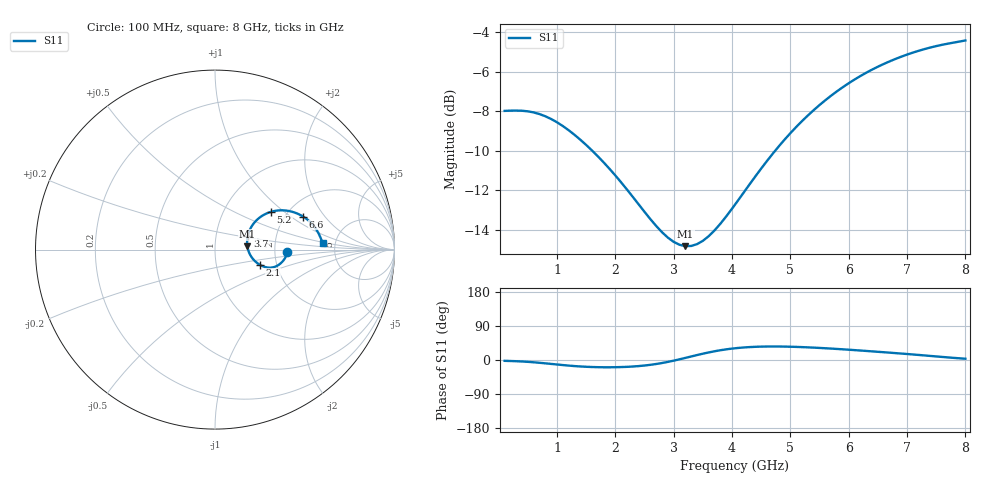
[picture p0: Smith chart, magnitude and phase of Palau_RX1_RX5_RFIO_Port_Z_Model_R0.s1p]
! Created Fri Jul 17 10:46:22 2020
! Palau RX1/RX5 RFIO Port Impedance Model.
! Revision		: R0.
! Impedance Mode 	: Balanced Differential-Mode.
! Impedance Format 	: Series Equivalent Differential Impedance (SEDZ).
# hz S ma R 50
! 1 Port Network Data from SP1.SP block
! freq  magS11  angS11
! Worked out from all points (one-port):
!   80 points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, 100 MHz to 8 GHz, reference 50 ohm
!   lowest |S11| = -14.8 dB at 3.2 GHz (marker M1), VSWR 1.44, Z = 72 + j2.62 ohm
!   |S11| at or under -10 dB: 1.604 GHz to 4.737 GHz (3.133 GHz wide, 98.8 % of centre)
!   S11 on the Smith chart (normalised r, x): 100 MHz: 2.32, -0.09; 2.1 GHz: 1.63, -0.29; 3.7 GHz: 1.43, +0.23; 5.2 GHz: 1.66, +0.81; 6.6 GHz: 2.48, +1.26; 8 GHz: 3.97, +0.44
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1e8  0.3991 -2.2
4e8  0.3994 -4.0
6e8  0.3955 -6.0
8e8  0.3867 -8.8
1.1e9  0.3653 -13.4
1.3e9  0.347 -16.0
1.6e9  0.3167 -18.5
1.8e9  0.2954 -19.2
2.1e9  0.2629 -18.6
2.4e9  0.2313 -16.0
2.8e9  0.1967 -7.9
3e9  0.186 -1.7
3.1e9  0.1829 1.9
3.2e9  0.1814 5.6
3.4e9  0.1836 13.1
3.5e9  0.1872 16.7
3.7e9  0.1989 23.1
4.1e9  0.2366 31.7
4.6e9  0.2983 35.6
5.1e9  0.3635 34.6
5.2e9  0.3762 34.0
5.6e9  0.4249 31.0
5.8e9  0.4476 29.1
6.1e9  0.4792 26.1
6.6e9  0.5247 20.5
7.1e9  0.5606 14.6
7.5e9  0.5822 9.4
8e9  0.6017 3.3
